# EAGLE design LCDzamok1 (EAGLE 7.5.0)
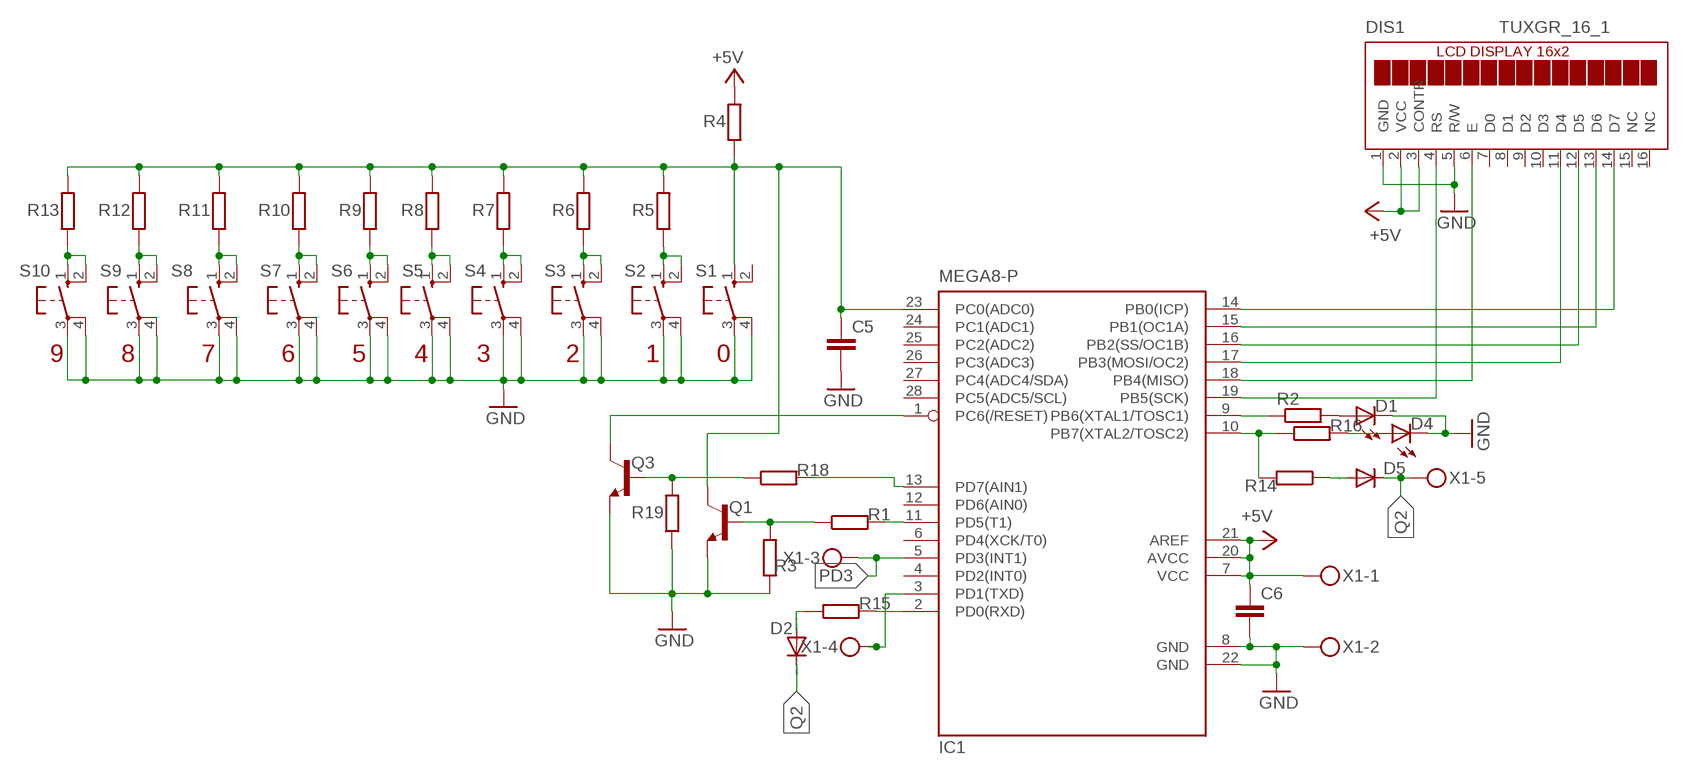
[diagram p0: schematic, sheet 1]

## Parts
C5  C-EUC1206  [C1206]
C6  C-EUC1206  [C1206]
D1  LED5MM  [LED5MM]
D2  1N4148DO35-7  [DO35-7]
D4  LED5MM  [LED5MM]
D5  1N4148DO35-10  [DO35-10]
DIS1  TUXGR_16_1  [TUXGR_16X1]
IC1  MEGA8-P  [DIL28-3]
Q1  BC337  [TO92]
Q3  BC337  [TO92]
R1  R-EU_0207/10  [0207/10]
R2  R-EU_0204/7  [0204/7]
R3  R-EU_M1206  [M1206]
R4  R-EU_0204/7  [0204/7]
R5  R-EU_M1206  [M1206]
R6  R-EU_M1206  [M1206]
R7  R-EU_M1206  [M1206]
R8  R-EU_M1206  [M1206]
R9  R-EU_M1206  [M1206]
R10  R-EU_M1206  [M1206]
R11  R-EU_M1206  [M1206]
R12  R-EU_M1206  [M1206]
R13  R-EU_M1206  [M1206]
R14  R-EU_0207/10  [0207/10]
R15  R-EU_0204/7  [0204/7]
R16  R-EU_M1206  [M1206]
R18  R-EU_0204/7  [0204/7]
R19  R-EU_M1206  [M1206]
S1  40-XX  [B3F-40XX]
S2  40-XX  [B3F-40XX]
S3  40-XX  [B3F-40XX]
S4  40-XX  [B3F-40XX]
S5  40-XX  [B3F-40XX]
S6  40-XX  [B3F-40XX]
S7  40-XX  [B3F-40XX]
S8  40-XX  [B3F-40XX]
S9  40-XX  [B3F-40XX]
S10  40-XX  [B3F-40XX]
X1  MKDSN1,5/5-5,08  [MKDSN1,5/5-5,08]

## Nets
+5V: C6.1 DIS1.2(VCC) DIS1.3(CONTR) IC1.7(VCC) IC1.20(AVCC) IC1.21(AREF) R4.2 X1.1
GND: C5.2 C6.2 D1.K(C) D4.K(C) DIS1.1(GND) DIS1.5(R/W) IC1.8(GND) IC1.22(GND) Q1.1(E) Q3.1(E) R3.1 R19.1 S1.3(P) S1.4(P1) S2.3(P) S2.4(P1) S3.3(P) S3.4(P1) S4.3(P) S4.4(P1) S5.3(P) S5.4(P1) S6.3(P) S6.4(P1) S7.3(P) S7.4(P1) S8.3(P) S8.4(P1) S9.3(P) S9.4(P1) S10.3(P) S10.4(P1) X1.2
N$1: DIS1.14(D7) IC1.14(PB0(ICP))
N$2: DIS1.13(D6) IC1.15(PB1(OC1A))
N$3: DIS1.12(D5) IC1.16(PB2(SS/OC1B))
N$4: DIS1.11(D4) IC1.17(PB3(MOSI/OC2))
N$5: DIS1.6(E) IC1.18(PB4(MISO))
N$6: DIS1.4(RS) IC1.19(PB5(SCK))
N$7: IC1.9(PB6(XTAL1/TOSC1)) R2.1
N$8: IC1.10(PB7(XTAL2/TOSC2)) R14.2 R16.1
N$9: D1.A R2.2
N$10: D4.A R16.2
N$11: IC1.2(PD0(RXD)) R15.2
N$12: D2.A R15.1
N$13: D5.A R14.1
N$14: IC1.3(PD1(TXD)) X1.4
N$15: C5.1 IC1.23(PC0(ADC0)) Q1.3(C) R4.1 R5.2 R6.2 R7.2 R8.2 R9.2 R10.2 R11.2 R12.2 R13.2 S1.1(S)
N$16: IC1.11(PD5(T1)) R1.2
N$17: Q1.2(B) R1.1 R3.2
N$18: IC1.13(PD7(AIN1)) R18.2
N$19: Q3.2(B) R18.1 R19.2
N$20: R13.1 S10.1(S) S10.2(S1)
N$22: R12.1 S9.1(S) S9.2(S1)
N$24: R11.1 S8.1(S) S8.2(S1)
N$26: R10.1 S7.1(S) S7.2(S1)
N$28: R9.1 S6.1(S) S6.2(S1)
N$30: R8.1 S5.1(S) S5.2(S1)
N$32: R7.1 S4.1(S) S4.2(S1)
N$34: R6.1 S3.1(S) S3.2(S1)
N$36: R5.1 S2.1(S) S2.2(S1)
PD3: IC1.5(PD3(INT1)) X1.3
Q2: D2.C D5.C X1.5
RESET: IC1.1(PC6(/RESET)) Q3.3(C)
Unconnected: DIS1.7(D0) DIS1.8(D1) DIS1.9(D2) DIS1.10(D3) DIS1.15(NC) DIS1.16(NC) IC1.4(PD2(INT0)) IC1.6(PD4(XCK/T0)) IC1.12(PD6(AIN0)) IC1.24(PC1(ADC1)) IC1.25(PC2(ADC2)) IC1.26(PC3(ADC3)) IC1.27(PC4(ADC4/SDA)) IC1.28(PC5(ADC5/SCL)) S1.2(S1)

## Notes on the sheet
- 9 | 8 | 7 | 6 | 5 | 4 | 3 | 2 | 1 | 0

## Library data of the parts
C5 C6 = rcl:C-EU: CAPACITOR, European symbol
D1 D4 = led:LED: LED
D2 D5 = diode:1N4148: DIODE
DIS1 = display-lcd:TUXGR_16_1: 1x16 LCD DISPLAY
IC1 = atmel:MEGA8-P: MICROCONTROLLER 8 Kbytes FLASH, 1 kbytes SRAM, 512 bytes EEPROM, USART, 4-channel 10 bit ADC, 2-channel 8 bit ADC Pin compatible with Atmega48, ATMega88, ATMega168 Source: avr.lbr; OC_FARNELL: unknown; OC_NEWARK: unknown
Q1 Q3 = transistor-neu-to92:BC337: NPN TRANSISTOR
R1-R16 R18 R19 = rcl:R-EU_: RESISTOR, European symbol
S1-S10 = switch-omron:40-XX: OMRON SWITCH; MF: OMRON COMPONENTS USA; MPN: B3F-4000; OC_FARNELL: 176434; OC_NEWARK: 36K3105
X1 = con-phoenix-508:MKDSN1,5/5-5,08: MKDSN 1,5/ 5-5,08 Printklemme Nennstrom: 13,5 A Nennspannung: 250 V Rastermaß: 5,08 mm Polzahl: 5 Anschlussart: Schraubanschluss Montage: Löten Anschlussrichtung Leiter/Platine: 0 ° Artikelnummer: 1729157 Source: http://eshop.phoenixcontact.com .. 1729157.pdf

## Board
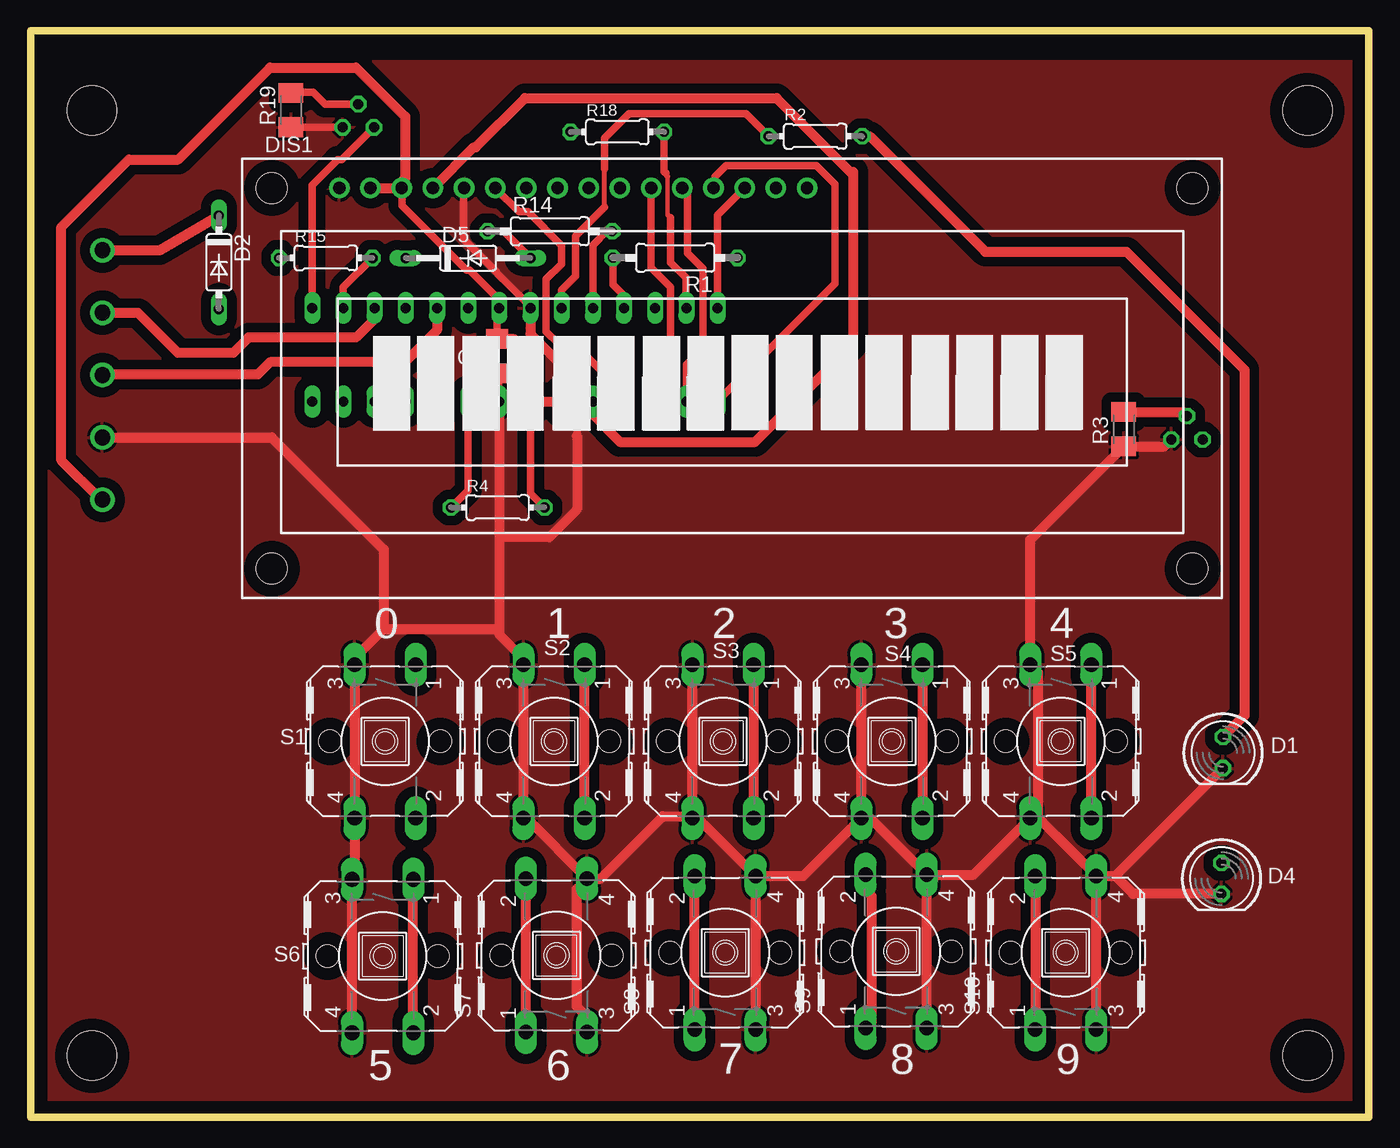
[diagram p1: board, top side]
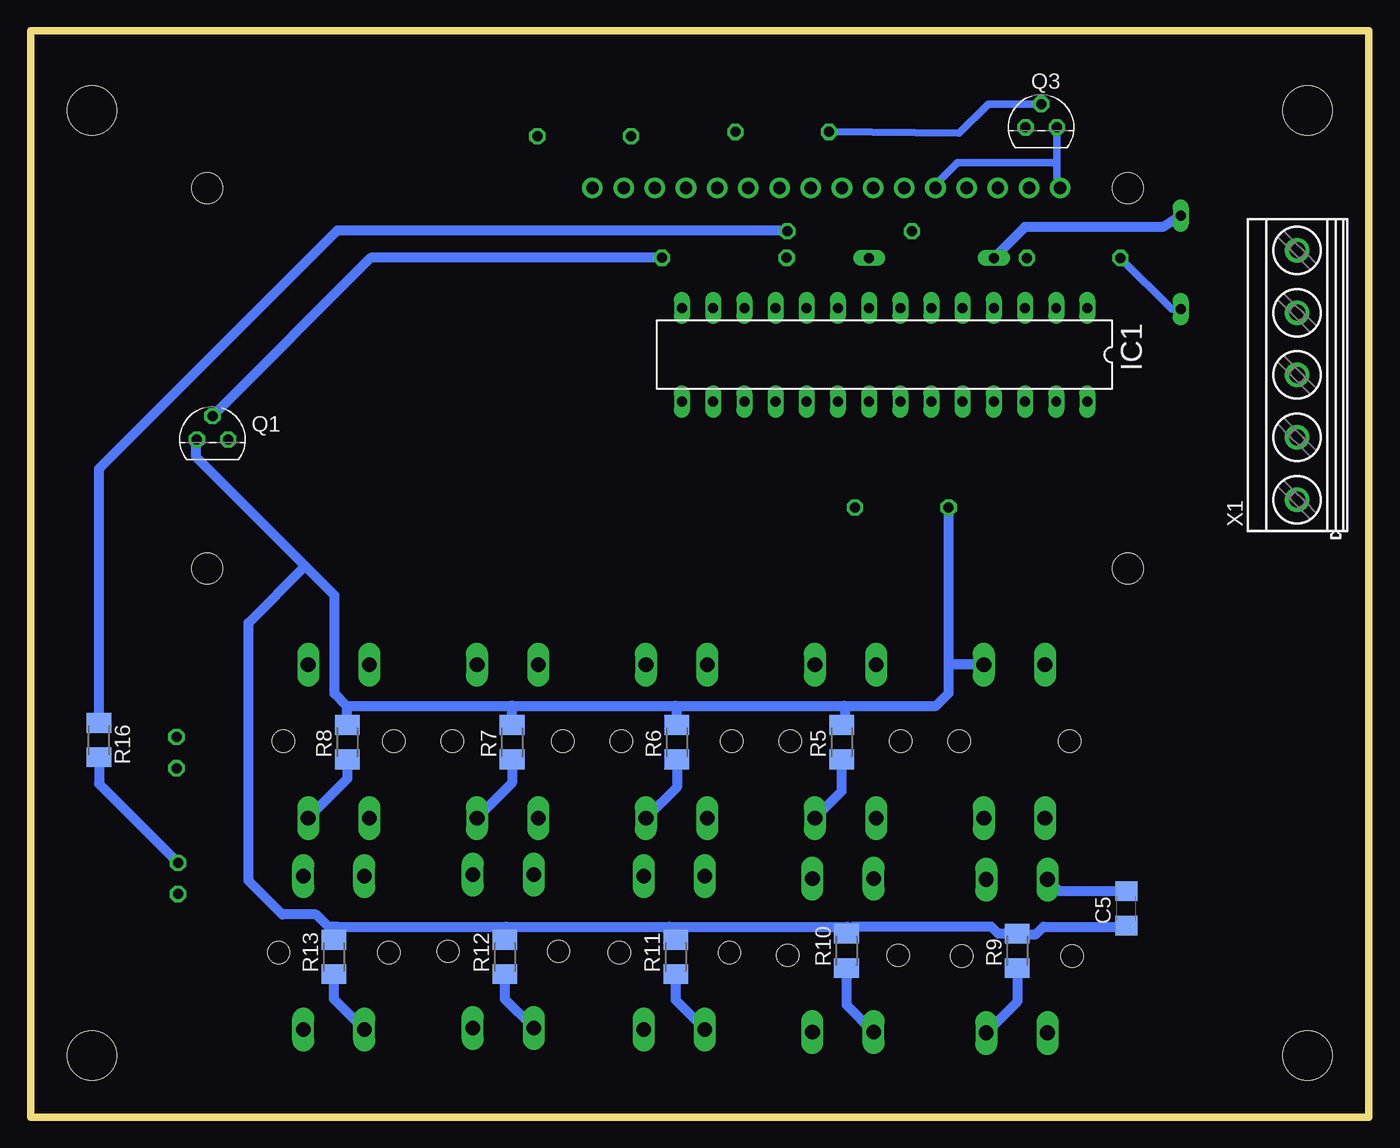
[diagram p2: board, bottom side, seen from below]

Size 109 x 88.5 mm. Coordinates in mm from the lower left corner, seen from the top.
Outline: 0,0 109,0 109,88.5 0,88.5 0,0
Copper layers (1*16): Top 0.035mm / dielectric 1.5mm / Bottom 0.035mm
Design rules "default": minimum track width 10mil, minimum drill 24mil, track to track 8mil, track to pad 8mil, pad to pad 8mil, via to via 8mil, smd to smd 8mil, copper to edge 40mil, drill to drill 8mil, minimum pad ring 10mil, minimum via ring 8mil, stop-mask expansion 4mil, vias tented up to drill 0mil, thermal gap 10mil
Holes 4 mm at 5,82 104,82 5,5 104,5

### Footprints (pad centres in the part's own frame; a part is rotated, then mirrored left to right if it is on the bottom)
C1206 = smd 1.6 x 1.8: 1 -1.4,0; 2 1.4,0
LED5MM = drill 0.813 octagon: A -1.27,0; K 1.27,0
DO35-7 = drill 0.813 long: A 3.81,0; C -3.81,0
DO35-10 = drill 0.813 long: A 5.08,0; C -5.08,0
TUXGR_16X1 = drill 1 pad 1.676: 1 -0.25,0.26; 2 2.29,0.26; 3 4.83,0.26; 4 7.37,0.26; 5 9.91,0.26; 6 12.45,0.26; 7 14.99,0.26; 8 17.53,0.26; 9 20.07,0.26; 10 22.61,0.26; 11 25.15,0.26; 12 27.69,0.26; 13 30.23,0.26; 14 32.77,0.26; 15 35.31,0.26; 16 37.85,0.26 | hole 2.5: -5.75,-30.74; 69.25,-30.74; -5.75,0.26; 69.25,0.26
DIL28-3 = drill 0.813 long: 1 -16.51,-3.81; 2 -13.97,-3.81; 3 -11.43,-3.81; 4 -8.89,-3.81; 5 -6.35,-3.81; 6 -3.81,-3.81; 7 -1.27,-3.81; 8 1.27,-3.81; 9 3.81,-3.81; 10 6.35,-3.81; 11 8.89,-3.81; 12 11.43,-3.81; 13 13.97,-3.81; 14 16.51,-3.81; 15 16.51,3.81; 16 13.97,3.81; 17 11.43,3.81; 18 8.89,3.81; 19 6.35,3.81; 20 3.81,3.81; 21 1.27,3.81; 22 -1.27,3.81; 23 -3.81,3.81; 24 -6.35,3.81; 25 -8.89,3.81; 26 -11.43,3.81; 27 -13.97,3.81; 28 -16.51,3.81
TO92 = drill 0.813 octagon: 1 1.27,0; 2 0,1.905; 3 -1.27,0
0207/10 = drill 0.813 octagon: 1 -5.08,0; 2 5.08,0
0204/7 = drill 0.813 octagon: 1 -3.81,0; 2 3.81,0
M1206 = smd 1.6 x 2: 1 -1.4,0; 2 1.4,0
B3F-40XX = drill 1.194 long: 1 -6.248,2.489; 2 6.248,2.489; 3 -6.248,-2.489; 4 6.248,-2.489 | hole 1.803: 0,-4.496; 0,4.496
MKDSN1,5/5-5,08 = drill 1.3 pad 2: 1 -10.181,0.025; 2 -5.101,0.025; 3 -0.021,0.025; 4 5.059,0.025; 5 10.139,0.025

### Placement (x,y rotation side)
C5  19.75,17 90 bottom
C6  38,62 270 top
D1  97.12,29.69 270 top
D2  15.33,69.63 270 top
D4  97,19.44 270 top
D5  35.62,69.98 0 top
DIS1  25.39,75.42 0 top
IC1  39.44,62.1 180 bottom
Q1  94.19,55.2 0 bottom
Q3  26.69,80.62 0 bottom
R1  52.5,70 180 top
R2  63.91,79.9 0 top
R3  89.04,56.04 90 top
R4  38.04,49.66 0 top
R5  42.95,30.54 90 bottom
R6  56.37,30.54 90 bottom
R7  69.79,30.54 90 bottom
R8  83.21,30.54 90 bottom
R9  28.63,13.54 90 bottom
R10  42.55,13.54 90 bottom
R11  56.47,13.04 90 bottom
R12  70.39,13.04 90 bottom
R13  84.31,13.04 90 bottom
R14  42.29,72.16 0 top
R15  24.04,69.99 0 top
R16  103.43,30.71 270 bottom
R18  47.79,80.25 0 top
R19  21.2,82.04 90 top
S1  28.87,30.61 270 top
S2  42.63,30.61 270 top
S3  56.39,30.61 270 top
S4  70.15,30.61 270 top
S5  83.91,30.61 270 top
S6  28.67,13.11 270 top
S7  42.83,13.17 90 top
S8  56.57,13.39 90 top
S9  70.5,13.5 90 top
S10  84.31,13.39 90 top
X1  5.82,60.47 90 bottom

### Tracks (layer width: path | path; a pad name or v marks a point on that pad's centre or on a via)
+5V
  Top 0.61: DIS1.3 30.25,75.65 30.25,74.25 35.5,69 35.75,69 38.17,66.58 IC1.7 38.09,65.91 38,66 C6.1 | IC1.21 40.71,50.8 R4.2
  Top 0.813: DIS1.2 DIS1.3 30,75.9 30,76 30.5,76.5 30.5,81.5 26.5,85.5 19.5,85.5 12,78 8,78 2.5,72.5 2.5,53.5 5.71,50.29 X1.1 | C6.1 38.02,63.38 39.38,63.38 40.71,62.04 IC1.21 IC1.20
GND
  Top 0.61: IC1.8 40.71,66.04 35.25,71.5 35.25,75.63 DIS1.5 | Q3.1 21.22,80.62 R19.1 | 44.5,60 44.5,55.5
  Top 0.813: C6.2 38,58.46 IC1.22 38.17,47.25 | 38.17,47.25 38.17,39.5 | 38.17,39.5 38.17,39.33 40,37.5 40,37 S2.3 S2.4 40.38,24.36 S7.4 | S7.4 46.42,19.42 51.5,24.5 53.76,24.5 S3.4 | S3.4 S3.3 | 26.5,18.75 26.38,18.87 S1.4 S1.3 26.38,37.38 28.75,39.75 29,39.75 | 26.5,18.75 26.5,19.04 S6.3 | S6.4 26.18,18.43 26.5,18.75 | S8.4 S8.3 | S3.4 54.34,24.36 S8.4 | S7.3 45.32,8.18 44.5,9 44.5,18.6 S7.4 | S4.4 S4.3 | S8.4 62.94,19.64 S4.4 | S4.4 68.38,24.36 S9.4 | S9.3 72.99,18.74 73.5,19.25 73.5,20 73.24,20 S9.4 | S9.4 76.81,19.75 S5.4 82.08,24.36 | S10.3 S10.4 | 82.08,24.36 S10.4 | S10.4 88.34,19.64 | 88.34,19.64 D1.K | 29,39.75 37.92,39.75 38.17,39.5 | X1.2 19.63,55.37 28.75,46.25 28.75,40 29,39.75 | D4.K 89.81,18.17 88.34,19.64 | Q1.1 92.36,54.64 R3.1 81.42,47.02 S5.3 82.08,36.2 82.08,24.36 | IC1.8 40.71,63.79 44.5,60 | 44.5,55.5 44.5,49.5 42.25,47.25 38.17,47.25
  Bottom 0.61: Q3.1 25.42,77.5 | 25.42,77.5 25.42,75.96 DIS1.1 | DIS1.5 35.3,75.95 33.5,77.75 25.67,77.75 25.42,77.5
  Bottom 0.813: C5.2 25.22,18.4 S6.3
  pour Top (isolate 0.8): 1.25,86 108,86 108,1 0.75,1 0.75,86
N$1
  Top 0.61: IC1.14 55.95,73.47 DIS1.14
N$2
  Top 0.61: IC1.15 55.95,58.33 65.5,67.88 65.5,76 64,77.5 56.62,77.5 55.75,76.62 55.75,75.81 DIS1.13
N$3
  Top 0.61: IC1.16 53.41,61.28 54.75,62.62 54.75,69.12 53.5,70.38 53.5,75.26 DIS1.12
N$4
  Top 0.61: DIS1.11 50.54,69.21 52.12,67.62 52.12,59.55 IC1.17
N$5
  Top 0.61: IC1.18 48.33,58.92 44.25,63 43,63 42,64 42,68.25 43.25,69.5 43.25,71 40.5,73.75 39.77,73.75 DIS1.6
N$6
  Top 0.813: IC1.19 45.79,57.21 48,55 59,55 67,63 67,76.75 | 67,76.75 67,77 | DIS1.4 36.08,79 36.25,79 40.25,83 60.75,83 67,76.75
N$7
  Top 0.406: 46.75,74.12 46.75,77.25
  Top 0.61: IC1.9 43.25,67.38 44.38,68.5 44.38,71.75 46.75,74.12 | 46.75,77.25 46.75,79.75 48.75,81.75 58.26,81.75 R2.1
N$8
  Top 0.61: IC1.10 45.79,71.04 47,72.25
  Top 0.813: 47,72.25 47.28,72.25 R14.2
  Bottom 0.813: R14.2 47.46,72.25 84,72.25 103.43,52.82 R16.1
N$9
  Top 0.813: R2.2 68.35,79.9 77.75,70.5 89.25,70.5 98.88,60.88 98.88,32.72 D1.A
N$10
  Bottom 0.813: R16.2 103.43,27.14 D4.A
N$11
  Top 0.61: IC1.2 25.47,67.61 R15.2
N$12
  Bottom 0.61: D2.A 16.06,65.82 R15.1
N$13
  Top 0.61: R14.1 38.52,72.16 D5.A
N$14
  Top 0.813: IC1.3 28.01,65.01 26.5,63.5 17.75,63.5 16.5,62.25 12,62.25 8.75,65.5 5.87,65.5 X1.4
N$15
  Top 0.61: IC1.23 35.63,51.05 R4.1
  Bottom 0.813: R5.2 42.64,32.25 42.64,33.39 42.75,33.5 | 42.75,33.5 35.25,33.5 34.23,34.52 34.23,36.75 | R6.2 56.37,33.37 56.5,33.5 | 56.5,33.5 42.75,33.5 | R7.2 69.79,33.46 | 69.79,33.46 69.75,33.5 56.5,33.5 | R8.2 83.21,33.46 83.25,33.5 | 83.25,33.5 69.83,33.5 69.79,33.46 | C5.1 19.85,15.5 26.5,15.5 27.1,14.9 28.59,14.9 R9.2 30.19,14.94 30.75,15.5 41.99,15.5 R10.2 42.5,14.99 42.5,15.5 57,15.5 | R12.2 70.39,15.36 70.25,15.5 | 70.25,15.5 57,15.5 | R11.2 56.47,14.97 57,15.5 | R13.2 84.31,15.19 84,15.5 | 84,15.5 70.25,15.5 | R4.1 34.23,36.75 | S1.1 34.12,36.86 34.23,36.75 | 83.25,33.5 84.25,34.5 84.25,42.5 86.62,44.88 | 86.62,44.88 95.5,53.75 95.5,55.16 Q1.3 | 84,15.5 84.75,15.5 85.75,16.5 88.5,16.5 91.25,19.25 91.25,40.25 86.62,44.88
N$16
  Top 0.61: R1.2 47.42,67.83 48.25,67 48.25,65.99 IC1.11
N$17
  Top 0.813: R3.2 93.86,57.44 Q1.2
  Bottom 0.813: R1.1 81.3,70 Q1.2
N$18
  Top 0.35: 51.88,76.62 51.88,73.5
  Top 0.406: 51.75,76.88 51.75,76.75 51.88,76.62 | 51.88,73.5 52.12,73.25
  Top 0.61: R18.2 51.6,77.03 51.75,76.88 | 52.12,73.25 52.12,69.62 53.38,68.38 53.38,65.94 IC1.13
N$19
  Top 0.61: Q3.2 23.98,82.53 23,83.5 21.26,83.5 R19.2
  Bottom 0.61: R18.1 33.37,80.13 31,82.5 26.71,82.5 Q3.2
N$20
  Top 0.813: S10.2 81.82,7.93 82.22,7.54 S10.1
  Bottom 0.813: R13.1 84.31,9.63 S10.1
N$22
  Top 0.813: S9.2 68.01,18.49 68.5,18 68.5,7.74 S9.1
  Bottom 0.813: R12.1 70.39,9.63 S9.1
N$24
  Top 0.813: S8.1 S8.2
  Bottom 0.813: R11.1 56.47,9.53 S8.1
N$26
  Top 0.813: S7.1 S7.2
  Bottom 0.813: R10.1 42.55,9.13 S7.1
N$28
  Top 0.813: S6.2 S6.1
  Bottom 0.813: R9.1 28.63,9.39 S6.2
N$30
  Top 0.813: S5.2 S5.1
  Bottom 0.813: R8.1 83.21,27.55 S5.2
N$32
  Top 0.813: S4.1 S4.2
  Bottom 0.813: R7.1 69.79,27.21 S4.2
N$34
  Top 0.813: S3.1 S3.2
  Bottom 0.813: R6.1 56.37,26.87 S3.2
N$36
  Top 0.813: S2.2 S2.1
  Bottom 0.813: R5.1 42.95,26.53 S2.2
PD3
  Top 0.813: IC1.5 33.09,64.09 30.5,61.5 19.5,61.5 18.5,60.5 5.9,60.5 X1.3
Q2
  Top 0.813: X1.5 10.5,70.61 D2.C
  Bottom 0.813: D5.C 28.02,72.5 16.77,72.5 D2.C
RESET
  Top 0.61: IC1.1 22.93,75.93 25,78 25.34,78 Q3.3

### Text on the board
tPlace: 0 | 1 | 2 | 3 | 4 | 7 | 8 | 9 | 5 | 6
